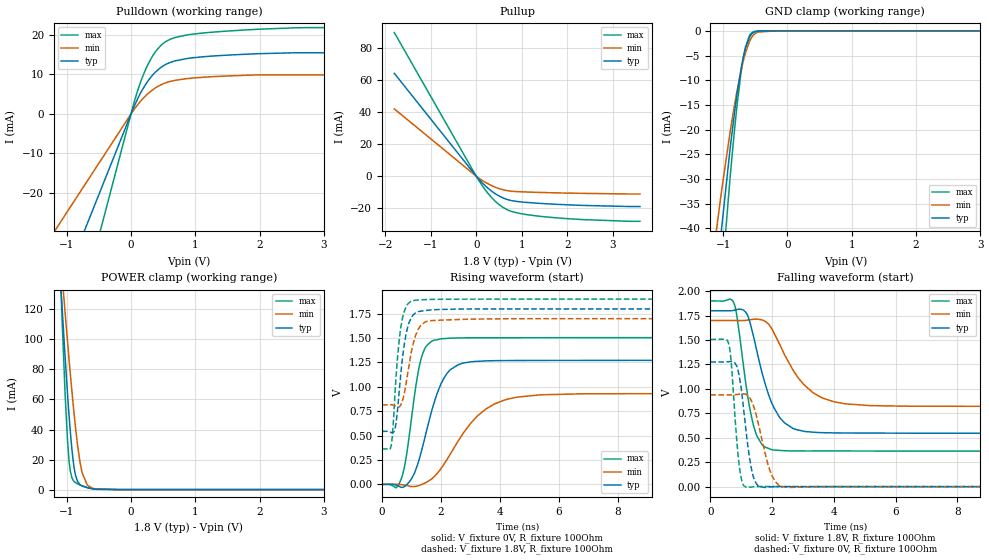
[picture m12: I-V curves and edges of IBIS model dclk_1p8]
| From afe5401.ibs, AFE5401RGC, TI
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|   dclk_1p8 Model
[Model]   dclk_1p8
Model_type   3-state
Polarity   Non-Inverting
Vmeas = 0.9
Vref = 0
Cref = 5pF
Rref = 100
|   typ   min   max
|   (nom PVT)   (fast PVT)   (slow PVT)
C_comp   1.702e-12   1.667e-12   1.738e-12
| Where nom  PVT is Nominal Process, 1.8V, 27C
|   Fast PVT is Strong Process,  1.9V, -40C
|   Slow PVT is Weak Process,   1.7V, 125C
[Voltage Range]   1.8   1.7   1.9
|Junction Temperature
[Temperature Range]   27   125   -40
[Pullup Reference]   1.8   1.7   1.9
[Pulldown Reference]   0   0   0
[Power Clamp Reference]   1.8   1.7   1.9
[GND Clamp Reference]   0   0   0
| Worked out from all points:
|   slope of the pulldown table from 0 to 0.27 V, typ, clamps not added: 31.9 ohm
|   slope of the pullup table from 0 to 0.27 V, typ, clamps not added: 34.6 ohm
|   GND clamp passes 1 mA (typ) near -0.58 V on its own axis
|   POWER clamp passes 1 mA (typ) near -0.65 V on its own axis
|   falling waveform, V_fixture 1.8V, R_fixture 100Ohm: 20-80 % time 695ps typ, 1.07ns min, 436ps max; typ from 1.8 V to 0.543 V
|   rising waveform, V_fixture 0V, R_fixture 100Ohm: 20-80 % time 725ps typ, 1.37ns min, 428ps max; typ from 0 V to 1.27 V
|   rising waveform, V_fixture 1.8V, R_fixture 100Ohm: 20-80 % time 284ps typ, 344ps min, 240ps max; typ from 0.543 V to 1.8 V
|   falling waveform, V_fixture 0V, R_fixture 100Ohm: 20-80 % time 300ps typ, 436ps min, 213ps max; typ from 1.27 V to 0 V
[Pulldown]
|   Voltage   I(typ)   I(min)   I(max)
-1.8V     -73.51mA   -44.92mA   -111.5mA
-84.3mV   -3.443mA   -2.104mA   -5.223mA
39.4mV    1.57mA     944.4uA    2.425mA
111.4mV   4.131mA    2.506mA    6.321mA
238.7mV   7.765mA    4.773mA    11.7mA
392.6mV   10.81mA    6.732mA    16.03mA
474.3mV   11.89mA    7.453mA    17.49mA
567mV     12.75mA    8.037mA    18.57mA
862.2mV   14.01mA    8.935mA    19.97mA
1.546V    14.93mA    9.65mA     21.03mA
2.561V    15.49mA    9.892mA    21.81mA
3.6V      15.49mA    9.892mA    21.85mA
[GND Clamp]
|   Voltage   I(typ)   I(min)   I(max)
-1.8V     -212.9mA   -134.6mA   -297.2mA
-1.179V   -61.16mA   -47.84mA   -78.13mA
-1.039V   -41.85mA   -33.74mA   -53.23mA
-1.023V   -39.8mA    -32.24mA   -50.56mA
-893.7mV  -24.06mA   -20.64mA   -29.93mA
-783.5mV  -12.78mA   -12.1mA    -15.04mA
-723.9mV  -7.858mA   -8.19mA    -8.642mA
-654.3mV  -3.57mA    -4.501mA   -3.344mA
-589.6mV  -1.253mA   -2.118mA   -897.7uA
-525.6mV  -316.4uA   -795.3uA   -160.9uA
-180mV    0A         -265.4nA   0A
3.6V      0A         0A         0A
[Pullup]
|   Voltage   I(typ)   I(min)   I(max)
-1.8V     64.38mA    42.09mA    89.94mA
34.2mV    -1.135mA   -725.1uA   -1.619mA
251.9mV   -7.372mA   -4.679mA   -10.53mA
411.7mV   -10.86mA   -6.845mA   -15.53mA
525.6mV   -12.77mA   -8.005mA   -18.3mA
682mV     -14.62mA   -9.077mA   -21.02mA
795.4mV   -15.43mA   -9.5mA     -22.27mA
1.329V    -16.93mA   -10.15mA   -24.93mA
2.345V    -18.34mA   -10.8mA    -27.24mA
3.6V      -19.05mA   -11.2mA    -28.29mA
[POWER Clamp]
|   Voltage   I(typ)   I(min)   I(max)
-1.8V     707.3mA    563.1mA    1.089A
-1.094V   138mA      154.9mA    139.7mA
-1.072V   121.9mA    143mA      114.2mA
-1.025V   88.52mA    117.9mA    64.1mA
-986.8mV  63.65mA    98.43mA    32.49mA
-964.8mV  50.36mA    87.47mA    19.92mA
-891mV    16.39mA    53.08mA    5.675mA
-834.4mV  5.687mA    30.78mA    3.916mA
-761.3mV  2.373mA    11.31mA    2.547mA
-678mV    1.244mA    2.861mA    1.321mA
-567mV    381.2uA    600.9uA    302.8uA
3.6V      0A         0A         0A
[Ramp]
R_load = 100
|   typ   min   max
dV/dt_r   0.764785/7.25167e-10  0.561073/1.35695e-09   0.903627/4.27837e-10
dV/dt_f   0.75417/6.91372e-10   0.529706/1.05813e-09   0.922272/4.34648e-10
[Falling Waveform]
V_fixture = 1.8V
V_fixture_min = 1.7V
V_fixture_max = 1.9V
R_fixture = 100Ohm
|   Time   V(typ)   V(min)   V(max)
0s        1.8V       1.7V       1.9V
765ps     1.804V     1.7V       1.878V
1.16ns    1.779V     1.702V     1.037V
1.395ns   1.544V     1.713V     632.4mV
1.66ns    1.185V     1.708V     437.2mV
2ns       849.9mV    1.611V     377.9mV
2.41ns    651.5mV    1.346V     367.2mV
3.055ns   564.9mV    1.037V     365.1mV
4.375ns   549mV      847.4mV    365.2mV
20ns      543.1mV    817.2mV    362.9mV
[Rising Waveform]
V_fixture = 0V
V_fixture_min = 0V
V_fixture_max = 0V
R_fixture = 100Ohm
|   Time   V(typ)   V(min)   V(max)
0s        1.023nV    76.16nV    424.3pV
650ps     -30.43mV   -2.64mV    53.74mV
825ps     -7.408mV   -10.64mV   289mV
1.29ns    287.8mV    -7.988mV   1.247V
1.765ns   835.7mV    77.64mV    1.478V
2.155ns   1.116V     231.5mV    1.495V
2.57ns    1.225V     437.6mV    1.502V
3.535ns   1.267V     774.8mV    1.503V
4.585ns   1.27V      894.7mV    1.503V
20ns      1.275V     935.1mV    1.506V
[Rising Waveform]
V_fixture = 1.8V
V_fixture_min = 1.7V
V_fixture_max = 1.9V
R_fixture = 100Ohm
|   Time   V(typ)   V(min)   V(max)
0s        543.4mV    815.6mV    363.2mV
310ps     531.8mV    817mV      396.3mV
425ps     558.2mV    806.5mV    861.1mV
545ps     825mV      792.4mV    1.367V
685ps     1.275V     851.1mV    1.691V
835ps     1.569V     1.076V     1.832V
1.06ns    1.738V     1.447V     1.885V
1.34ns    1.778V     1.639V     1.893V
1.85ns    1.793V     1.683V     1.898V
20ns      1.8V       1.7V       1.9V
[Falling Waveform]
V_fixture = 0V
V_fixture_min = 0V
V_fixture_max = 0V
R_fixture = 100Ohm
|   Time   V(typ)   V(min)   V(max)
0s        1.275V     939.7mV    1.506V
610ps     1.279V     938.7mV    1.449V
935ps     1.136V     946.2mV    223.7mV
1.045ns   891.5mV    949.8mV    34.79mV
1.185ns   495.6mV    939.1mV    -11.6mV
1.37ns    130mV      850.2mV    -1.908mV
1.54ns    11.33mV    665.4mV    1.788mV
1.94ns    -1.903mV   157.8mV    1.091mV
2.325ns   1.458mV    -2.769mV   445.8uV
20ns      166.3nV    654.3nV    -89.18nV
